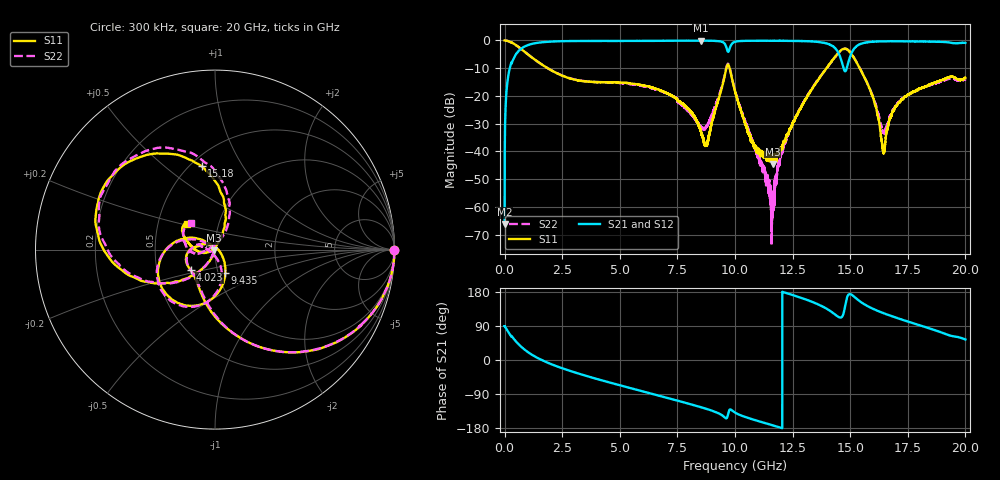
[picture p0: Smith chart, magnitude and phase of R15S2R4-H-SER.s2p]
!{R15S2R4}
!Johanson Technology Inc.
!www.johansontechnology.com
!Test Board Conditions:
!Substrate Type  RO4350B
!Substrate Thickness  20 mil
!Substrate Dk  3.66
!TL Type: GCPW
!TL Trace Width  34 mil
!TL Gap  10 mil
!Electrode orientation  Horizontal
!DUT TOPOLOGY	SERIES
!Mounting Pad LxW  26x52 mil
! Created Sat Feb  6 13:51:02 2021
# hz S ma R 50
! 2 Port Network Data from SP1.SP block
! freq  magS11  angS11  magS21  angS21  magS12  angS12  magS22  angS22
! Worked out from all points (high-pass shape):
!   20001 points, 300 kHz to 20 GHz, reference 50 ohm
!   highest |S21| = -0.07 dB at 8.504 GHz (marker M1); lowest = -66.3 dB at 300 kHz (marker M2)
!   |S21| within 3 dB of the highest: 704.1 MHz to 9.647 GHz (8.943 GHz wide, 173 % of centre); 15.16 GHz to end of sweep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
!   lowest |S11| = -44.5 dB at 11.63 GHz (marker M3), VSWR 1.01, Z = 49.6 - j0.391 ohm
!   |S11| at or under -10 dB: 1.869 GHz to 9.626 GHz (7.756 GHz wide, 135 % of centre); 9.767 GHz to 13.97 GHz (4.203 GHz wide, 35.4 % of centre); 15.41 GHz to end of sweep
!   |S22| runs from -74.2 to 0.0 dB; largest |S21 - S12| = 0.013
!   S11 on the Smith chart (normalised r, x): 300 kHz: open; 4.023 GHz: 0.74, -0.17; 9.435 GHz: 1.08, -0.29; 15.18 GHz: 0.57, +0.68; 20 GHz: 0.70, +0.21
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300000  1 -0.3  0.0004849 89.1  0.0004413 91.5  0.997 -0.1
1.293e8  0.9809 -12.7  0.1886 76.9  0.1894 77.0  0.9809 -12.7
4.663e8  0.8392 -38.9  0.5404 50.8  0.5414 50.9  0.8373 -38.9
1.4893e9  0.3989 -86.7  0.9134 3.5  0.9137 3.5  0.3986 -86.1
3.3343e9  0.1865 -128.6  0.9787 -38.1  0.9787 -38.2  0.1882 -126.7
4.0233e9  0.1774 -140.3  0.9804 -50.4  0.9789 -50.4  0.1776 -139.6
6.6673e9  0.1304 177.0  0.9845 -93.5  0.9858 -93.5  0.1278 175.6
8.5043e9  0.02386 112.1  0.9924 -124.3  0.9904 -124.3  0.02828 -155.7
8.7813e9  0.01356 29.1  0.9878 -129.4  0.9894 -129.3  0.02844 -106.6
9.4353e9  0.1429 -66.5  0.9454 -145.7  0.948 -145.6  0.1515 -75.6
9.7043e9  0.367 -140.6  0.6215 -141.7  0.6248 -141.6  0.3774 -140.2
1.00003e10  0.1211 148.7  0.946 -138.6  0.9467 -138.7  0.1257 153.5
1.07823e10  0.01466 158.0  0.986 -156.9  0.987 -156.9  0.01397 125.8
1.16303e10  0.005933 -138.4  0.9865 -172.3  0.9866 -172.3  0.001629 -165.8
1.21903e10  0.01556 -108.9  0.9837 177.4  0.9832 177.5  0.01458 -116.9
1.33343e10  0.1321 -123.8  0.9606 153.8  0.9625 153.8  0.1346 -124.2
1.46363e10  0.6826 167.3  0.4092 113.4  0.4115 113.2  0.6695 164.1
1.51803e10  0.4703 99.2  0.7218 166.6  0.7109 166.6  0.4774 94.8
1.60313e10  0.08224 64.5  0.9507 133.9  0.9489 134.0  0.08607 59.9
1.64203e10  0.01056 121.1  0.9664 124.3  0.9611 124.2  0.02267 110.5
1.66673e10  0.03225 -161.4  0.9688 118.5  0.9627 118.7  0.03621 175.6
2e10  0.2128 137.7  0.9036 54.1  0.8975 53.9  0.199 131.5
